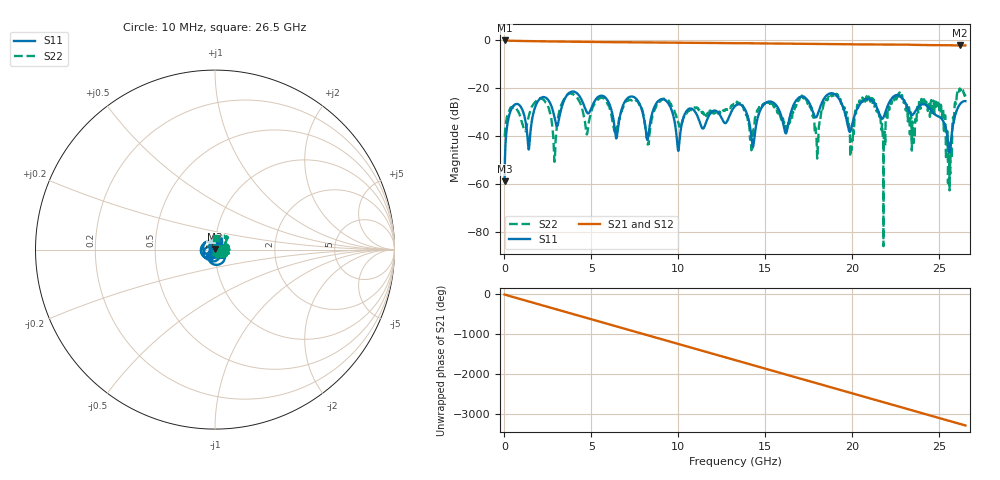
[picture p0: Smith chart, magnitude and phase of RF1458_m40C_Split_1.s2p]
!Keysight Technologies,N5245B,MY55451909,A.13.80.08
!Automatic Fixture Removal (AFR)
!Date: Thursday, August 27, 2020, 03:55:23
!S2P File: Measurements: S11,S21,S12,S22:
# MHz S  RI  R 50
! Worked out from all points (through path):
!   2650 points, 10 MHz to 26.5 GHz, reference 50 ohm
!   highest |S21| = 0.00 dB at 10 MHz (marker M1); lowest = -2.1 dB at 26.18 GHz (marker M2)
!   group delay of S21, straight-line fit = 345 ps
!   lowest |S11| = -58.7 dB at 10 MHz (marker M3), VSWR 1.00, Z = 50 + j0.115 ohm
!   |S11| at or under -10 dB: start of sweep to end of sweep
!   |S22| runs from -85.8 to -20.0 dB; largest |S21 - S12| = 1.5e-15
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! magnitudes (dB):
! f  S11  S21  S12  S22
! 10 MHz  -58.7  0.0  0.0  -39.7
! 580 MHz  -26.8  -0.2  -0.2  -27.7
! 1.4 GHz  -45.5  -0.3  -0.3  -31.5
! 2.09 GHz  -24.0  -0.4  -0.4  -24.2
! 2.88 GHz  -32.2  -0.4  -0.4  -50.6
! 3.54 GHz  -23.4  -0.5  -0.5  -23.2
! 4.43 GHz  -24.7  -0.6  -0.6  -27.6
! 6.44 GHz  -40.9  -0.8  -0.8  -36.5
! 7.53 GHz  -24.0  -0.8  -0.8  -24.7
! 8.25 GHz  -40.9  -0.8  -0.8  -43.3
! 8.84 GHz  -25.3  -0.9  -0.9  -26.0
! 10 GHz  -46.0  -0.9  -0.9  -34.2
! 13.26 GHz  -27.4  -1.2  -1.2  -25.6
! 14.22 GHz  -41.4  -1.2  -1.2  -44.9
! 17.67 GHz  -28.5  -1.4  -1.4  -29.7
! 19.08 GHz  -23.0  -1.6  -1.6  -22.5
! 19.96 GHz  -36.1  -1.6  -1.6  -45.3
! 22.09 GHz  -26.3  -1.7  -1.7  -27.6
! 24.98 GHz  -31.8  -2.0  -2.0  -26.0
! 25.61 GHz  -46.1  -2.0  -2.0  -49.9
! 26.18 GHz  -26.7  -2.1  -2.1  -20.0
! 26.5 GHz  -25.3  -2.1  -2.1  -23.9
